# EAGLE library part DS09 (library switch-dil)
DIL/CODE SWITCH
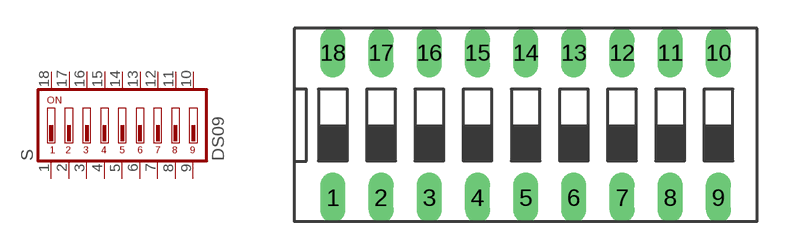
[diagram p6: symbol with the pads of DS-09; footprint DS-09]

Designator prefix S

## DS09 (MPN: MCDS09; OC_FARNELL: 1255227; OC_NEWARK: 26M1107)  [DS-09]
1  1  pas
2  2  pas
3  3  pas
4  4  pas
5  5  pas
6  6  pas
7  7  pas
8  8  pas
9  9  pas
10  10  pas
11  11  pas
12  12  pas
13  13  pas
14  14  pas
15  15  pas
16  16  pas
17  17  pas
18  18  pas

## Footprint DS-09 (pad centres in mm)
DIL/CODE SWITCH Mors distributor Buerklin, 17G564
drill 0.813 long: 1 -10.16,-3.81; 2 -7.62,-3.81; 3 -5.08,-3.81; 4 -2.54,-3.81; 5 0,-3.81; 6 2.54,-3.81; 7 5.08,-3.81; 8 7.62,-3.81; 9 10.16,-3.81; 10 10.16,3.81; 11 7.62,3.81; 12 5.08,3.81; 13 2.54,3.81; 14 0,3.81; 15 -2.54,3.81; 16 -5.08,3.81; 17 -7.62,3.81; 18 -10.16,3.81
